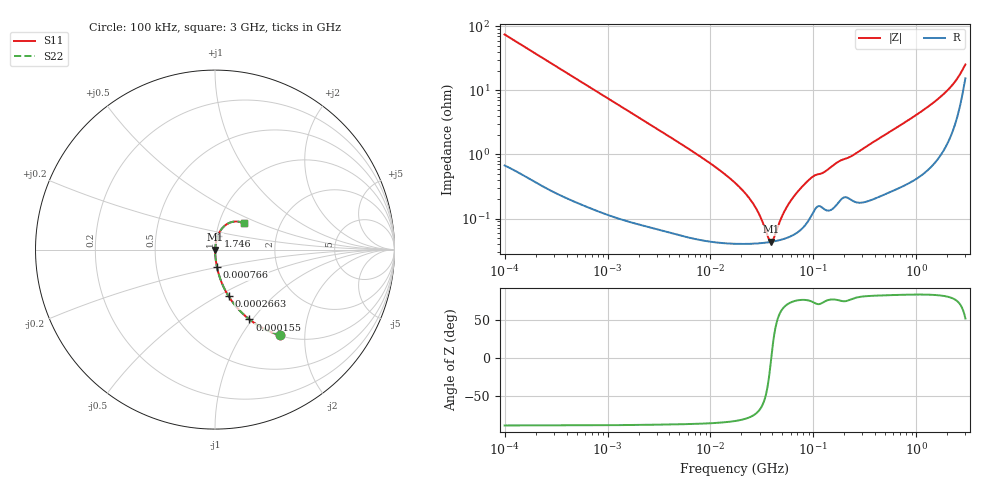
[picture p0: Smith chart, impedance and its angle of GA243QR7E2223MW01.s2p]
!Murata Part Number: GA243QR7E2223MW01
!These Parameters are Measured in Series Mode Connection
!Data Generated on Jun 19, 2026
!  o--ll--o
!Port1  Port2
!  o------o
!Operation Temp=25[degC], DC Bias Voltage=0[V]
!Freq. Start=100[kHz] Stop=3[GHz] 401[Steps]
# Hz S RI R 50
!Freq.(Hz) S11(Real) S11(Imag) S21(Real) S21(Imag) S12(Real) S12(Imag) S22(Real) S22(Imag)
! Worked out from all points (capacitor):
!   401 points, 100 kHz to 3 GHz, reference 50 ohm
!   read as one part in series: C = 21.3 nF near 105.3 kHz
!   lowest |Z| = 43.3 mohm at 38.51 MHz (marker M1)
!   series resonance near 38.99 MHz, so ESL is about 780 pH
!   S11 on the Smith chart (normalised r, x): 100 kHz: 1.01, -1.49; 155 kHz: 1.01, -0.97; 266.3 kHz: 1.01, -0.56; 766 kHz: 1.00, -0.20; 1.746 GHz: 1.02, +0.16; 3 GHz: 1.31, +0.40
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100000  0.3595 -0.4754  0.6405 0.4754  0.6405 0.4754  0.3595 -0.4754
154981  0.1918 -0.389  0.8082 0.389  0.8082 0.389  0.1918 -0.389
266273  0.0761 -0.2601  0.9239 0.2601  0.9239 0.2601  0.0761 -0.2601
562235  0.0192 -0.1314  0.9808 0.1314  0.9808 0.1314  0.0192 -0.1314
766005  0.0109 -0.0975  0.9891 0.0975  0.9891 0.0975  0.0109 -0.0975
3161081  0.00124 -0.024  0.9988 0.024  0.9988 0.024  0.00124 -0.024
9574722  0.000496 -0.00757  0.9995 0.00757  0.9995 0.00757  0.000496 -0.00757
1.77727e7  0.000414 -0.00345  0.9996 0.00345  0.9996 0.00345  0.000414 -0.00345
2.684345e7  0.000408 -0.00152  0.9996 0.00152  0.9996 0.00152  0.000408 -0.00152
3.053531e7  0.000412 -0.000982  0.9996 0.000982  0.9996 0.000982  0.000412 -0.000982
3.657227e7  0.000425 -0.000255  0.9996 0.000255  0.9996 0.000255  0.000425 -0.000255
3.850681e7  0.00043 -4.9e-05  0.9996 4.9e-05  0.9996 4.9e-05  0.00043 -4.9e-05
4.160216e7  0.00044 0.00026  0.9996 -0.00026  0.9996 -0.00026  0.00044 0.00026
4.982709e7  0.000472 0.000995  0.9995 -0.000995  0.9995 -0.000995  0.000472 0.000995
5.967813e7  0.000527 0.00177  0.9995 -0.00177  0.9995 -0.00177  0.000527 0.00177
7.525761e7  0.000671 0.00288  0.9993 -0.00288  0.9993 -0.00288  0.000671 0.00288
9.738194e7  0.00118 0.00426  0.9988 -0.00426  0.9988 -0.00426  0.00118 0.00426
2.400085e8  0.00198 0.0094  0.998 -0.0094  0.998 -0.0094  0.00198 0.0094
5.475153e8  0.00304 0.0221  0.997 -0.0221  0.997 -0.0221  0.00304 0.0221
1.746113e9  0.0162 0.0784  0.9838 -0.0784  0.9838 -0.0784  0.0162 0.0784
2.441062e9  0.0501 0.1295  0.9499 -0.1295  0.9499 -0.1295  0.0501 0.1295
3e9  0.1592 0.1464  0.8408 -0.1464  0.8408 -0.1464  0.1592 0.1464
